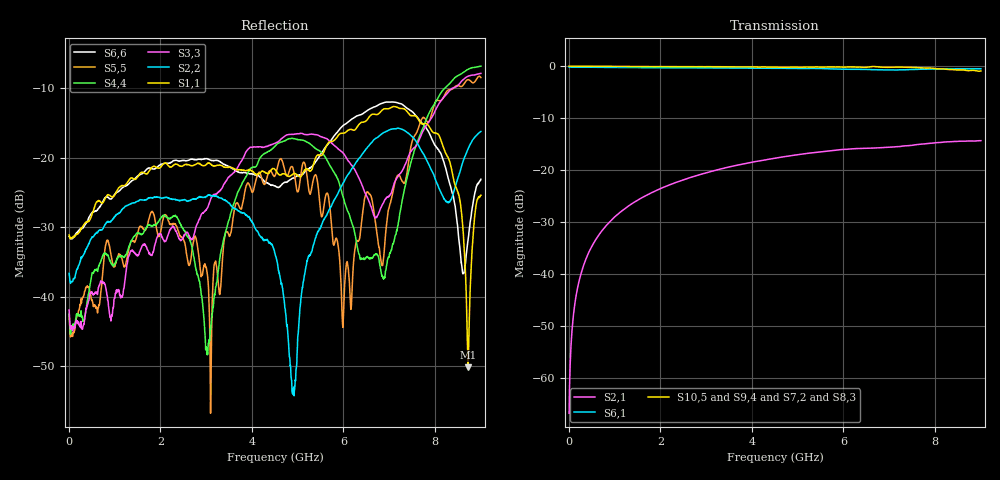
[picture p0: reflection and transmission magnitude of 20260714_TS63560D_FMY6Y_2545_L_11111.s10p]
# GHz S DB R 50
! CMT, SN0916, 25263762, 26.7.0
! Date: 15.07.2026 13:51:31
! Data: Format
! Freq S1.1:dB/Ang S1.2:dB/Ang S1.3:dB/Ang S1.4:dB/Ang S1.5:dB/Ang S1.6:dB/Ang S1.7:dB/Ang S1.8:dB/Ang S1.9:dB/Ang S1.10:dB/Ang
!  S2.1:dB/Ang S2.2:dB/Ang S2.3:dB/Ang S2.4:dB/Ang S2.5:dB/Ang S2.6:dB/Ang S2.7:dB/Ang S2.8:dB/Ang S2.9:dB/Ang S2.10:dB/Ang
!  S3.1:dB/Ang S3.2:dB/Ang S3.3:dB/Ang S3.4:dB/Ang S3.5:dB/Ang S3.6:dB/Ang S3.7:dB/Ang S3.8:dB/Ang S3.9:dB/Ang S3.10:dB/Ang
!  S4.1:dB/Ang S4.2:dB/Ang S4.3:dB/Ang S4.4:dB/Ang S4.5:dB/Ang S4.6:dB/Ang S4.7:dB/Ang S4.8:dB/Ang S4.9:dB/Ang S4.10:dB/Ang
!  S5.1:dB/Ang S5.2:dB/Ang S5.3:dB/Ang S5.4:dB/Ang S5.5:dB/Ang S5.6:dB/Ang S5.7:dB/Ang S5.8:dB/Ang S5.9:dB/Ang S5.10:dB/Ang
!  S6.1:dB/Ang S6.2:dB/Ang S6.3:dB/Ang S6.4:dB/Ang S6.5:dB/Ang S6.6:dB/Ang S6.7:dB/Ang S6.8:dB/Ang S6.9:dB/Ang S6.10:dB/Ang
!  S7.1:dB/Ang S7.2:dB/Ang S7.3:dB/Ang S7.4:dB/Ang S7.5:dB/Ang S7.6:dB/Ang S7.7:dB/Ang S7.8:dB/Ang S7.9:dB/Ang S7.10:dB/Ang
!  S8.1:dB/Ang S8.2:dB/Ang S8.3:dB/Ang S8.4:dB/Ang S8.5:dB/Ang S8.6:dB/Ang S8.7:dB/Ang S8.8:dB/Ang S8.9:dB/Ang S8.10:dB/Ang
!  S9.1:dB/Ang S9.2:dB/Ang S9.3:dB/Ang S9.4:dB/Ang S9.5:dB/Ang S9.6:dB/Ang S9.7:dB/Ang S9.8:dB/Ang S9.9:dB/Ang S9.10:dB/Ang
!  S10.1:dB/Ang S10.2:dB/Ang S10.3:dB/Ang S10.4:dB/Ang S10.5:dB/Ang S10.6:dB/Ang S10.7:dB/Ang S10.8:dB/Ang S10.9:dB/Ang S10.10:dB/Ang
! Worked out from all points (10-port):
!   2001 points, 10 MHz to 9 GHz, reference 50 ohm
!   strongest paths, dB at 10 MHz, 2.257 GHz, 4.505 GHz, 6.753 GHz, 9 GHz:
!     S10,5: -0.1, -0.2, -0.2, -0.2, -1.0
!     S9,4: -0.1, -0.2, -0.4, -0.4, -1.5
!     S7,2: -0.1, -0.3, -0.4, -0.6, -0.6
!     S8,3: -0.1, -0.2, -0.4, -0.4, -1.3
!     S6,1: -0.3, -0.4, -0.5, -0.7, -0.6
!     S2,1: -66.7, -22.7, -17.7, -15.7, -14.4
!   lowest |S11| = -50.1 dB at 8.721 GHz (marker M1), VSWR 1.01, Z = 49.9 + j0.286 ohm
!   |S11| at or under -10 dB: start of sweep to end of sweep
